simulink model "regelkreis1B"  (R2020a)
settings: Solver=ode45  StartTime=0.0  StopTime=10  MaxStep=0.01  RelTol=1e-3  EnableMultiTasking=on
libraries: libregler1 x2

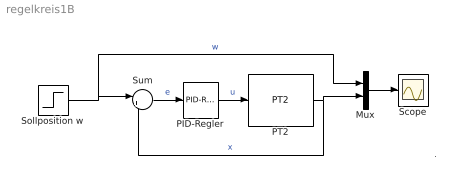
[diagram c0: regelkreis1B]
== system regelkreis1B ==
  note: .
  Mux : Mux  Inputs=2
  PID-Regler : libregler1/PID-Regler  Kp=10  Ki=20  Kd=5
  PT2 : libregler1/PT2  D=0.2  om0=3  b0=1.0
  Scope : Scope
  Sollposition w : Step  SampleTime=0
  Sum : Sum  Inputs=|+-  SaturateOnIntegerOverflow=on
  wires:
  PID-Regler/1 -> PT2/1  "u"
  PT2/1 -> Sum/2, Mux/2  "x"
  Sollposition w/1 -> Sum/1, Mux/1  "w"
  Sum/1 -> PID-Regler/1  "e"
  Mux/1 -> Scope/1
